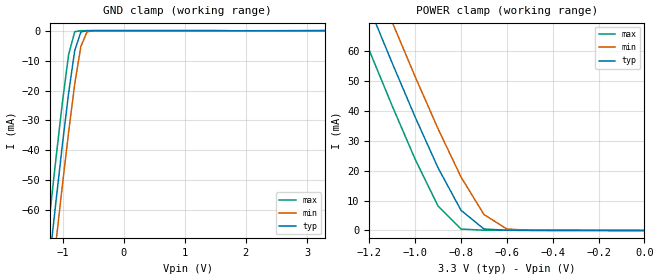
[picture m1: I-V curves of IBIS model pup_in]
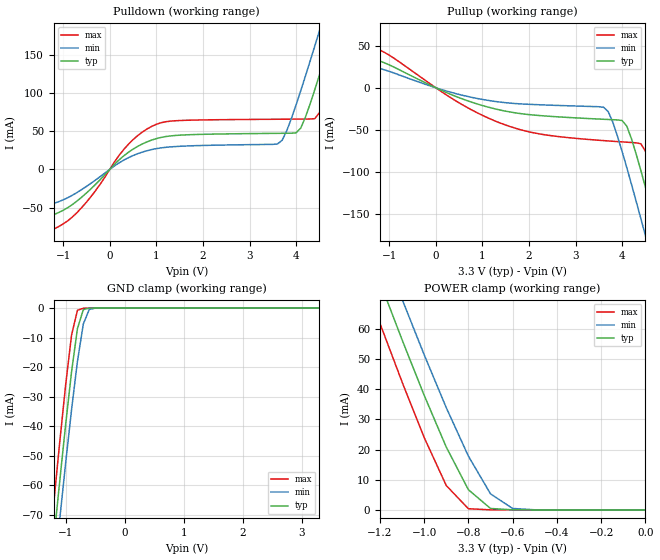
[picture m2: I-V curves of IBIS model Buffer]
| IBIS file EG2002_L.ibs
[IBIS ver]   2.1
[File name]   eg2002_l.ibs
[File Rev]   2
[Date]   December 26, 2006
[Source]   Hspice simulation by NPC using CF5032 schematics
[Disclaimer]   Data is for modeling purpose only and is not guaranteed.
[Copyright]   Epson Toyocom Corp.
|   Component EG-2002CA (62.5M - 80.0MHz)
[Component]   EG-2002CA
[Manufacturer]   Epson Toyocom Corp.
[Package]
| variable   typ   min   max
R_pkg   0.913   NA   NA
L_pkg   2.00nH   NA   NA
C_pkg   3.36pF   NA   NA
[Pin]  signal_name   model_name   R_pin   L_pin   C_pin
1   oe   pup_in   NA   NA   NA
2   vss   GND   NA   NA   NA
3   out   Buffer   NA   NA   NA
4   vdd   POWER   NA   NA   NA
| Models and submodels in the file (2): pup_in (Input), Buffer (3-state)
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|   Model pup_in
[Model]   pup_in
Model_type   Input
Polarity   Non-Inverting
C_comp   0.412pF  0.385pF  0.444pF
Vinl = 0.99V | VIL = VCC * 0.3
Vinh = 2.31V | VIH = VCC * 0.7
|   typ   min   max
[Temperature Range]   25.00  70.00  0.00
[Voltage Range]   3.30V  3.00V  3.60V
[POWER Clamp Reference]   3.30V  3.00V  3.60V
[GND Clamp Reference]   0.00V  0.00V  0.00V
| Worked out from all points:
|   GND clamp passes 1 mA (typ) near -0.71 V on its own axis
|   POWER clamp passes 1 mA (typ) near -0.71 V on its own axis
[GND_clamp]
| voltage = voutput
| voltage   I(typ)   I(min)   I(max)
-3.3V     -484.7mA   -497.3mA   -471.6mA
-1.3V     -93.15mA   -106.8mA   -78.84mA
-1.2V     -74.31mA   -87.99mA   -59.94mA
-1.1V     -55.78mA   -69.45mA   -41.42mA
-1V       -37.78mA   -51.32mA   -23.67mA
-900mV    -20.84mA   -33.88mA   -8.024mA
-800mV    -6.686mA   -17.84mA   -381.4uA
-700mV    -463.3uA   -5.315mA   -14.29uA
-600mV    -16.01uA   -459.9uA   -11.51uA
-500mV    -6.034uA   -22.38uA   -11.49uA
3.3V      3.292pA    13.43uA    -31.97uA
[POWER_clamp]
| voltage = vcc - voutput
| voltage   I(typ)   I(min)   I(max)
-3.3V     485mA      497.5mA    472.1mA
-1.3V     93.24mA    106.9mA    78.99mA
-1.2V     74.39mA    88.04mA    60.07mA
-1.1V     55.85mA    69.5mA     41.55mA
-1V       37.85mA    51.34mA    23.76mA
-900mV    20.88mA    33.92mA    8.114mA
-800mV    6.74mA     17.85mA    467uA
-700mV    507.6uA    5.336mA    88.25uA
-600mV    53.76uA    484.2uA    72.65uA
-500mV    36.05uA    42.36uA    59.98uA
0V        3.292pA    4.769pA    3.573pA
|   Model Buffer
[Model] Buffer
Model_type   3-state
Polarity   Non-Inverting
Enable   Active-High
C_comp   0.412pF  0.385pF  0.444pF
|   typ   min   max
[Temperature Range]   25.00  70.00  0.00
[Voltage Range]   3.30V  3.00V  3.60V
[POWER Clamp Reference]   3.30V  3.00V  3.60V
[GND Clamp Reference]   0.00V  0.00V  0.00V
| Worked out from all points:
|   slope of the pulldown table from 0 to 0.495 V, typ, clamps not added: 18.9 ohm
|   slope of the pullup table from 0 to 0.495 V, typ, clamps not added: 42.4 ohm
|   GND clamp passes 1 mA (typ) near -0.71 V on its own axis
|   POWER clamp passes 1 mA (typ) near -0.71 V on its own axis
[Pulldown]
|   voltage = vcc - voutput
|   voltage   I(typ)   I(min)   I(max)
-3.3V     -67.9mA    -55.9mA    -80.8mA
-1.1V     -56.56mA   -42.35mA   -74.95mA
-500mV    -30.9mA    -22.28mA   -42.88mA
400mV     22.32mA    15.26mA    32.79mA
1V        40.24mA    27.14mA    58.95mA
3.6V      47.15mA    33.22mA    65.58mA
3.8V      47.26mA    50.7mA     65.67mA
4.1V      54.11mA    103mA      65.8mA
4.5V      123.3mA    181.1mA    74.07mA
4.8V      183.2mA    241.9mA    128.1mA
5.1V      245.2mA    303.7mA    189.6mA
6.6V      571mA      623.8mA    524.1mA
[Pullup]
|   voltage = vcc -voutput
|   voltage   I(typ)   I(min)   I(max)
-3.3V     56.1mA     44.5mA     69.8mA
-1.4V     35.8mA     26mA       50.1mA
500mV     -11.79mA   -7.945mA   -17.92mA
1.5V      -27.84mA   -17.78mA   -44.33mA
3.6V      -37.48mA   -23.17mA   -62.84mA
3.8V      -37.99mA   -41.07mA   -63.63mA
4.1V      -45.68mA   -95.02mA   -64.74mA
4.4V      -98.06mA   -155.2mA   -66.53mA
4.5V      -118.2mA   -175.8mA   -75.32mA
4.8V      -180.6mA   -238.4mA   -132.9mA
5V        -223.2mA   -280.6mA   -175.6mA
6.6V      -571mA     -622.6mA   -530.7mA
[GND_clamp]
|   voltage = voutput
|   voltage   I(typ)   I(min)   I(max)
-3.3V     -526.8mA   -531.7mA   -523.8mA
-1.3V     -98.82mA   -111.1mA   -86.63mA
-1.2V     -78.5mA    -91.12mA   -65.77mA
-1.1V     -58.64mA   -71.55mA   -45.45mA
-1V       -39.49mA   -52.56mA   -26.11mA
-900mV    -21.66mA   -34.48mA   -9.195mA
-800mV    -6.961mA   -18.06mA   -743.7uA
-700mV    -519.1uA   -5.372mA   -64.86uA
-600mV    -19.87uA   -469.5uA   -6.162uA
-500mV    -1.463uA   -21.54uA   -440.7nA
3.3V      12.1pA     29.59nA    9.014pA
[POWER_clamp]
|   voltage = vcc - voutput
|   voltage   I(typ)   I(min)   I(max)
-3.3V     520.8mA    523.7mA    523.9mA
-1.3V     95.28mA    108.3mA    81.98mA
-1.2V     75.68mA    88.98mA    61.95mA
-1.1V     56.51mA    69.97mA    42.51mA
-1V       38.04mA    51.5mA     24.05mA
-900mV    20.85mA    33.91mA    8.076mA
-800mV    6.683mA    17.84mA    373.3uA
-700mV    456.7uA    5.311mA    2.878uA
-600mV    10.2uA     456.6uA    20.85nA
-500mV    208.7nA    19.2uA     171.7pA
0V        12.1pA     53.26pA    10.82pA
[Ramp]
| variable   typ   min   max
dV/dt_r   0.897/347p   0.583/413p   1.273/260p
dV/dt_f   1.089/438p   0.761/509p   1.417/355p
R_load = 50.000
| End [Model] Buffer
| End [Component] EG-2002CA
